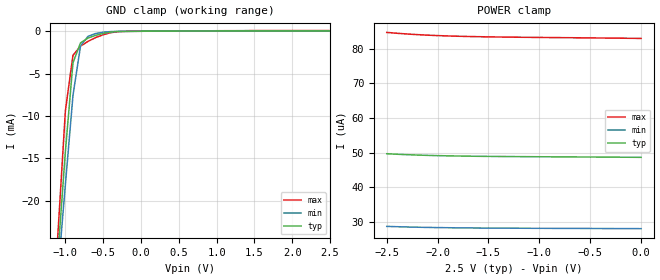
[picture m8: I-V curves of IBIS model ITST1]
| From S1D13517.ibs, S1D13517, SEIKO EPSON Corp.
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[Model]   ITST1
Model_type Input
C_comp   5p   4p   6p
[Temperature Range] 50   100   0
[Voltage Range]   2.5   2.3   2.7
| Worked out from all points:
|   GND clamp passes 1 mA (typ) near -0.74 V on its own axis
[GND Clamp]
-2.5V     -207.7mA   -184.5mA   -240.2mA
-1.1V     -26.51mA   -28.73mA   -24.05mA
-1V       -14.18mA   -18.09mA   -9.388mA
-900mV    -3.728mA   -7.591mA   -2.846mA
-800mV    -1.374mA   -1.731mA   -1.756mA
-700mV    -794.5uA   -595.6uA   -1.191mA
-600mV    -479.5uA   -268.1uA   -750uA
-500mV    -252.1uA   -112.2uA   -406.9uA
-300mV    -28.29uA   -13.68uA   -46.34uA
2.5V      48.61uA    27.99uA    82.94uA
[POWER Clamp]
-2.5V     49.65uA    28.63uA    84.76uA
-2.4V     49.5uA     28.53uA    84.51uA
-2.3V     49.38uA    28.45uA    84.3uA
-2.2V     49.27uA    28.39uA    84.12uA
-2.1V     49.18uA    28.33uA    83.97uA
-2V       49.1uA     28.28uA    83.84uA
-1.9V     49.04uA    28.24uA    83.74uA
-1.7V     48.95uA    28.18uA    83.58uA
-1.5V     48.88uA    28.13uA    83.47uA
-1.3V     48.83uA    28.1uA     83.39uA
-300mV    48.66uA    28uA       83.11uA
0V        48.61uA    27.97uA    83.02uA
